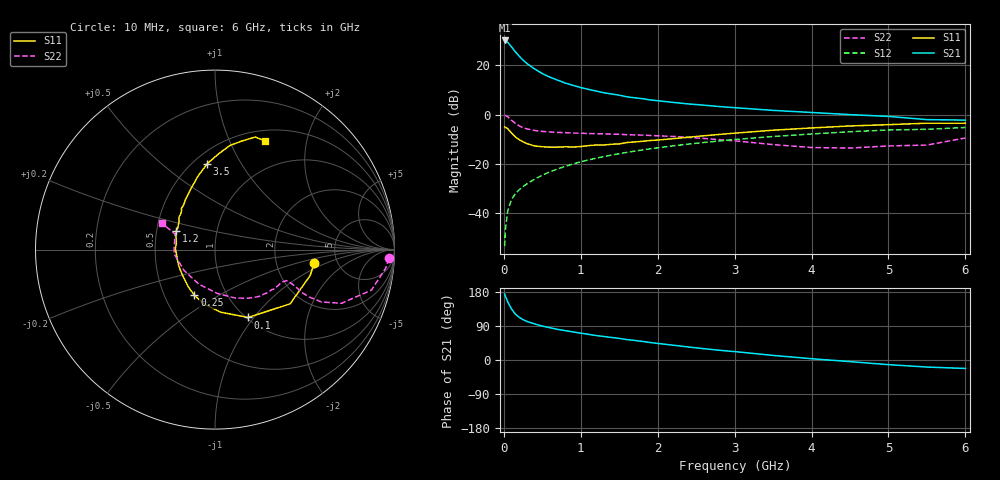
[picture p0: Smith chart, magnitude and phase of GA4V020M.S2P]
! Infineon Technologies  Discrete & RF Semiconductors
! BF775
! Si NPN RF Bipolar Junction Transistor in SOT23
! VCE = 4 V  IC = 20 mA
! Common Emitter S-Parameters:  May  1996
# GHz  S  MA  R  50
!  f  S11  S21  S12  S22
! GHz  MAG  ANG  MAG  ANG  MAG  ANG  MAG  ANG
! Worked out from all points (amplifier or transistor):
!   36 points, 10 MHz to 6 GHz, reference 50 ohm
!   highest |S21| = 30.1 dB at 10 MHz (marker M1)
!   |S21| within 3 dB of that: start of sweep to 109.6 MHz
!   unconditionally stable (mu >= 1): 397 MHz to 2.944 GHz
!   at 250 MHz: K = 0.86, MSG = 25.7 dB, |S12| = -29.3 dB
!   at 1.4 GHz: K = 1.11, MAG = 10.5 dB, |S12| = -16.5 dB
!   at 6 GHz: K = 0.94, MSG = 1.5 dB, |S12| = -5.3 dB
!   S11 on the Smith chart (normalised r, x): 10 MHz: 3.35, -0.72; 100 MHz: 1.02, -0.94; 250 MHz: 0.71, -0.39; 1.2 GHz: 0.63, +0.14; 3.5 GHz: 0.58, +0.73; 6 GHz: 0.63, +1.37
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0.01  0.5578 -7.6  32.13 174.1  0.0021 91.0  0.9707 -2.9
0.02  0.5496 -15.2  31.6 168.5  0.0045 82.8  0.9576 -6.1
0.05  0.5162 -35.8  29.45 153.6  0.0109 75.8  0.9007 -14.5
0.1  0.4207 -64.0  23.78 134.5  0.0188 68.7  0.7657 -23.0
0.15  0.3499 -85.0  18.86 121.1  0.0246 66.5  0.6607 -26.2
0.2  0.3088 -101.6  15.37 112.6  0.0295 66.4  0.5872 -26.7
0.25  0.2789 -114.3  12.77 106.4  0.0342 66.8  0.5403 -26.3
0.3  0.2564 -125.1  10.92 101.8  0.0389 68.1  0.5131 -25.3
0.4  0.2295 -142.9  8.459 95.2  0.0487 69.2  0.4737 -24.1
0.5  0.2215 -155.7  6.804 89.4  0.0583 70.4  0.4538 -23.6
0.6  0.2167 -165.3  5.755 85.2  0.0684 70.4  0.4427 -23.5
0.8  0.2212 178.6  4.363 77.3  0.0885 69.9  0.4276 -24.4
1  0.2236 165.1  3.54 70.8  0.1093 69.2  0.4179 -25.9
1.1  0.2331 159.5  3.247 67.8  0.1191 68.2  0.4103 -27.5
1.2  0.2401 154.0  3.006 64.5  0.1294 67.5  0.4068 -28.5
1.6  0.2695 138.2  2.293 53.8  0.1699 63.8  0.3886 -34.8
2.2  0.3226 120.8  1.767 39.1  0.2307 57.5  0.359 -46.5
2.8  0.3937 106.6  1.454 25.7  0.2903 50.5  0.3077 -61.5
3.5  0.4803 95.2  1.215 12.1  0.3572 41.5  0.2446 -86.8
4.5  0.5855 81.9  0.996 -4.3  0.447 28.2  0.208 -145.7
5.5  0.6662 70.3  0.788 -18.6  0.5007 13.0  0.2395 158.7
6  0.6662 65.2  0.77 -22.3  0.5458 8.9  0.3333 153.4
